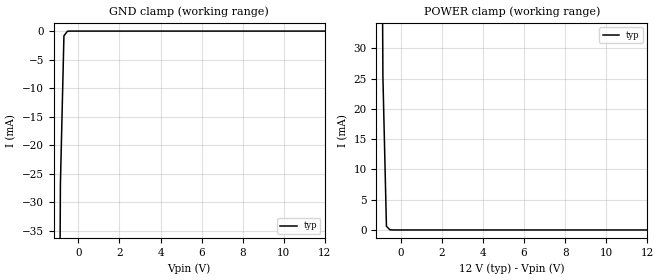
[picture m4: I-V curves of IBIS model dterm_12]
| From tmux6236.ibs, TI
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| dterm_12
[Model]   dterm_12
Model_type   Terminator
|   typ   min   max
C_comp   2.533030e-11   NA   NA
[Voltage Range]   12   NA   NA
[Temperature Range]   27   NA   NA
[Power Clamp Reference]   12   NA   NA
[GND Clamp Reference]   0   NA   NA
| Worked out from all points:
|   GND clamp passes 1 mA (typ) near -0.71 V on its own axis
|   POWER clamp passes 1 mA (typ) near -0.71 V on its own axis
[GND Clamp]
|   Voltage   I(typ)   I(min)   I(max)
-5V       -7.828A    NA         NA
-1.051V   -137.9mA   NA         NA
-878.8mV  -26.8mA    NA         NA
-707.1mV  -828.8uA   NA         NA
-535.4mV  -21.42uA   NA         NA
12V       5.312nA    NA         NA
[POWER Clamp]
|   Voltage   I(typ)   I(min)   I(max)
-5V       10.13A     NA         NA
-1.05V    133.2mA    NA         NA
-878.8mV  25.28mA    NA         NA
-707.1mV  609.3uA    NA         NA
-535.4mV  25.46uA    NA         NA
12V       -4.959nA   NA         NA
